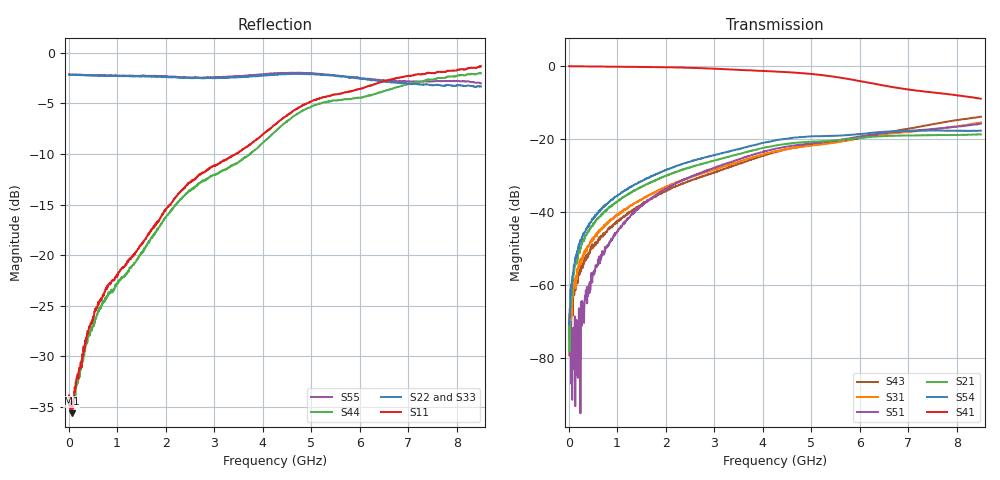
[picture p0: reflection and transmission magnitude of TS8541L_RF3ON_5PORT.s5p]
! Created with skrf (http://scikit-rf.org).
# Hz S RI R 50.0
!freq ReS11 ImS11 ReS12 ImS12 ReS13 ImS13
! ReS14 ImS14 ReS15 ImS15
! ReS21 ImS21 ReS22 ImS22 ReS23 ImS23
! ReS24 ImS24 ReS25 ImS25
! ReS31 ImS31 ReS32 ImS32 ReS33 ImS33
! ReS34 ImS34 ReS35 ImS35
! ReS41 ImS41 ReS42 ImS42 ReS43 ImS43
! ReS44 ImS44 ReS45 ImS45
! ReS51 ImS51 ReS52 ImS52 ReS53 ImS53
! ReS54 ImS54 ReS55 ImS55
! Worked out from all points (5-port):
!   1601 points, 10 MHz to 8.5 GHz, reference 50 ohm
!   strongest paths, dB at 10 MHz, 2.132 GHz, 4.255 GHz, 6.378 GHz, 8.5 GHz:
!     S41: -0.2, -0.5, -1.6, -5.1, -9.1
!     S54: -70.2, -27.9, -20.5, -18.2, -17.8
!     S21: -70.3, -29.5, -21.9, -19.4, -18.8
!     S51: -72.7, -32.8, -22.8, -18.6, -15.9
!     S31: -79.4, -32.5, -23.5, -19.0, -15.6
!     S43: -71.3, -33.5, -23.7, -18.8, -14.0
!   lowest |S11| = -35.6 dB at 63.06 MHz (marker M1), VSWR 1.03, Z = 51.6 - j0.58 ohm
!   |S11| at or under -10 dB: start of sweep to 3.444 GHz
